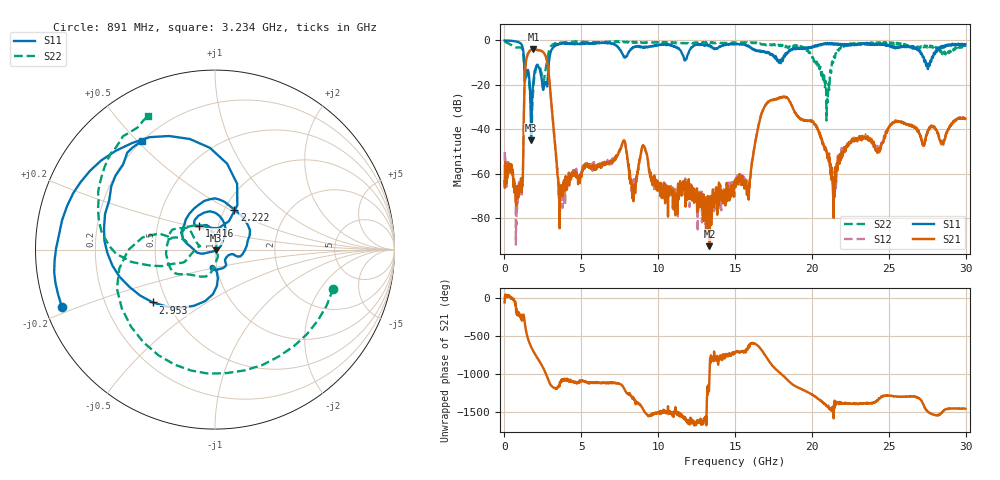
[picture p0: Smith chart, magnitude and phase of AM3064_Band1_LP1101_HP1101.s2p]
# Hz S DB R 50.0
!freq dBS11 angS11 dBS21 angS21 dBS12 angS12 dBS22 angS22
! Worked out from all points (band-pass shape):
!   1600 points, 10 MHz to 29.98 GHz, reference 50 ohm
!   highest |S21| = -3.98 dB at 1.884 GHz (marker M1); lowest = -92.7 dB at 13.34 GHz (marker M2)
!   |S21| within 3 dB of the highest: 1.478 GHz to 2.671 GHz (1.193 GHz wide, 57.5 % of centre)
!   lowest |S11| = -45.0 dB at 1.734 GHz (marker M3), VSWR 1.01, Z = 50.3 - j0.443 ohm
!   |S11| at or under -10 dB: 1.277 GHz to 2.889 GHz (1.612 GHz wide, 77.4 % of centre); 17.95527 GHz to 17.98551 GHz (30.24 MHz wide, 0.168 % of centre); 27.4 GHz to 27.68 GHz (282.9 MHz wide, 1.03 % of centre)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
!   |S22| runs from -41.9 to -0.4 dB; largest |S21 - S12| = 0.01
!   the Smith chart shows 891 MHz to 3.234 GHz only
!   S11 on the Smith chart (normalised r, x): 891 MHz: 0.05, -0.18; 1.416 GHz: 0.81, +0.22; 2.222 GHz: 1.11, +0.53; 2.953 GHz: 0.42, -0.31; 3.234 GHz: 0.20, +0.52
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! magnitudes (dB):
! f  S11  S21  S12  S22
! 10 MHz  0.0  -63.3  -50.3  -0.4
! 891 MHz  -0.8  -70.8  -69.9  -3.2
! 1.116 GHz  -1.9  -66.9  -70.6  -3.5
! 1.416 GHz  -16.0  -8.8  -8.8  -15.7
! 1.734 GHz  -45.0  -4.3  -4.2  -31.9
! 1.884 GHz  -18.5  -4.0  -4.0  -20.8
! 2.222 GHz  -12.1  -4.5  -4.3  -11.6
! 2.953 GHz  -6.9  -20.4  -20.3  -3.6
! 3.234 GHz  -2.7  -42.7  -42.5  -1.6
! 3.646 GHz  -1.6  -69.1  -66.9  -1.0
! 5.015 GHz  -1.4  -60.1  -59.1  -0.6
! 7.751 GHz  -7.3  -45.1  -45.3  -0.7
! 10 GHz  -2.1  -66.1  -64.7  -0.9
! 13.34 GHz  -2.2  -92.7  -76.8  -1.2
! 15 GHz  -1.7  -64.2  -63.2  -1.3
! 15.87 GHz  -2.3  -65.4  -65.4  -0.9
! 17.18 GHz  -5.4  -27.7  -27.4  -2.1
! 19.99 GHz  -3.3  -36.5  -36.4  -6.9
! 20.98 GHz  -1.3  -51.5  -50.5  -26.4
! 21.42 GHz  -1.7  -79.9  -67.8  -7.7
! 25 GHz  -2.1  -39.4  -39.3  -1.2
! 29.98 GHz  -1.8  -35.3  -35.3  -2.9
